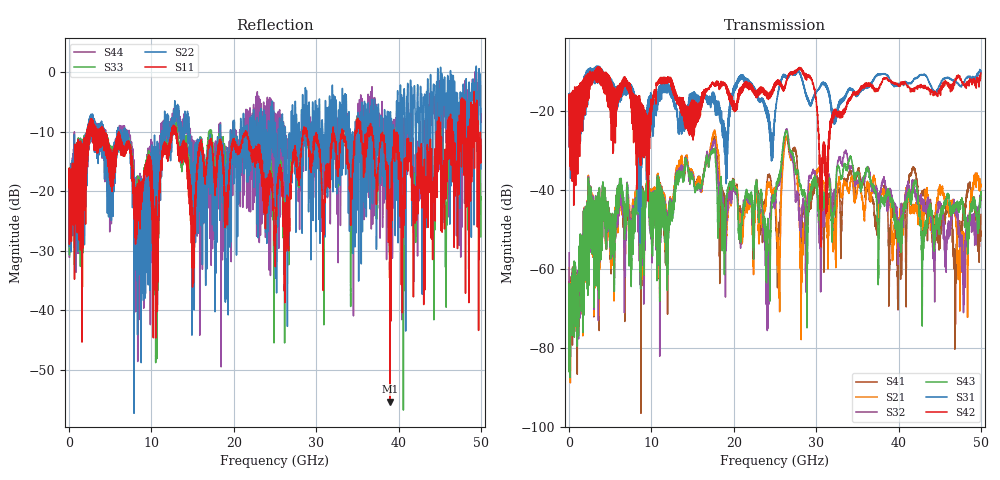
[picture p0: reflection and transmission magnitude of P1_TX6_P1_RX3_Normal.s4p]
!Keysight Technologies,N5225B,MY57041031,A.13.20.10
!Date: Friday, May 31, 2019 11:17:39
!Correction: S11(Full 4 Port(1,2,3,4))
!S12(Full 4 Port(1,2,3,4))
!S13(Full 4 Port(1,2,3,4))
!S14(Full 4 Port(1,2,3,4))
!S21(Full 4 Port(1,2,3,4))
!S22(Full 4 Port(1,2,3,4))
!S23(Full 4 Port(1,2,3,4))
!S24(Full 4 Port(1,2,3,4))
!S31(Full 4 Port(1,2,3,4))
!S32(Full 4 Port(1,2,3,4))
!S33(Full 4 Port(1,2,3,4))
!S34(Full 4 Port(1,2,3,4))
!S41(Full 4 Port(1,2,3,4))
!S42(Full 4 Port(1,2,3,4))
!S43(Full 4 Port(1,2,3,4))
!S44(Full 4 Port(1,2,3,4))
!S4P File: Measurements: <S11,S12,S13,S14>,
!<S21,S22,S23,S24>,
!<S31,S32,S33,S34>,
!<S41,S42,S43,S44>:
# Hz S  dB  R 50.0
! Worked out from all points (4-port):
!   5000 points, 10 MHz to 50 GHz, reference 50 ohm
!   strongest paths, dB at 10 MHz, 12.51 GHz, 25.01 GHz, 37.51 GHz, 50 GHz:
!     S42: -19.6, -14.3, -13.3, -14.7, -10.5
!     S31: -19.4, -15.5, -21.6, -10.8, -9.9
!     S43: -75.4, -45.8, -41.1, -53.1, -40.9
!     S32: -56.0, -44.8, -44.2, -41.2, -41.0
!     S21: -59.7, -44.0, -41.6, -48.1, -39.1
!     S41: -63.3, -44.5, -44.0, -48.5, -46.3
!   lowest |S11| = -55.4 dB at 38.96 GHz (marker M1), VSWR 1.00, Z = 50.1 + j0.0941 ohm
!   |S11| at or under -10 dB: 4.286 GHz to 12.47 GHz (8.179 GHz wide, 97.6 % of centre); 13.02 GHz to 21.43 GHz (8.403 GHz wide, 48.8 % of centre); 21.46 GHz to 28.42 GHz (6.96 GHz wide, 27.9 % of centre)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
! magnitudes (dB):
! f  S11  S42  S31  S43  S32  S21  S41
! 10 MHz  -19.4  -19.6  -19.4  -75.4  -56.0  -59.7  -63.3
! 17.53 GHz  -14.7  -13.0  -16.7  -30.2  -28.0  -25.6  -26.9
! 24.08 GHz  -19.5  -16.3  -20.9  -50.6  -59.0  -39.1  -37.6
! 26.36 GHz  -23.7  -13.0  -11.8  -25.1  -24.7  -26.8  -26.9
! 28.25 GHz  -12.0  -9.9  -12.0  -40.8  -45.2  -63.5  -48.7
! 38.96 GHz  -55.4  -12.4  -12.3  -41.7  -40.4  -43.4  -52.5
! 50 GHz  -11.3  -10.5  -9.9  -40.9  -41.0  -39.1  -46.3
